|-- THIS SOFTWARE IS PROVIDED BY FREESCALE "AS IS" AND ANY EXPRESSED OR
|-- IMPLIED WARRANTIES, INCLUDING, BUT NOT LIMITED TO, THE IMPLIED WARRANTIES
|-- OF MERCHANTABILITY AND FITNESS FOR A PARTICULAR PURPOSE ARE DISCLAIMED.
|-- IN NO EVENT SHALL FREESCALE OR ITS CONTRIBUTORS BE LIABLE FOR ANY DIRECT,
|-- INDIRECT, INCIDENTAL, SPECIAL, EXEMPLARY, OR CONSEQUENTIAL DAMAGES
|-- (INCLUDING, BUT NOT LIMITED TO, PROCUREMENT OF SUBSTITUTE GOODS OR
|-- SERVICES; LOSS OF USE, DATA, OR PROFITS; OR BUSINESS INTERRUPTION)
|-- HOWEVER CAUSED AND ON ANY THEORY OF LIABILITY, WHETHER IN CONTRACT,
|-- STRICT LIABILITY, OR TORT (INCLUDING NEGLIGENCE OR OTHERWISE) ARISING
|-- IN ANY WAY OUT OF THE USE OF THIS SOFTWARE, EVEN IF ADVISED OF
|-- THE POSSIBILITY OF SUCH DAMAGE.
[IBIS Ver]   5.0
[Comment Char] |_char
[File name]   k10_120_144mbga_full.ibs
[File Rev]   1.2
[Date]   12/03/2013
[Source]   Freescale, MSG, MCD, Design
[Notes]   IBIS model for K10 microprocessor covers 1.71 - 3.6V range
[Disclaimer]   The model given below represents 144MBGA package on K10 family
[Copyright]   Copyright, Freescale, Inc., 2013
|  Component K10
[Component]   K10
[Manufacturer]  Freescale, Inc.
[Package]
|   typ   min   max
R_pkg   0.10565   0.037083   0.19461
L_pkg   2.143e-9   8.357e-10   4.07e-9
C_pkg   1.414e-12   1.006e-12   2.364e-12
[Pin]   Signal_name   model_name   R_pin   L_pin   C_pin
E5   VDD   POWER
E6   VDD   POWER
E7   VDD   POWER
E8   VDD   POWER
H5   VDDA   POWER
F5   VDD   POWER
F8   VDD   POWER
L6   VBAT   POWER
J3   ADC0SE16   NC   0.10508   2.028e-9   1.342e-12
K3   ADC1SE16   NC   0.11747   2.367e-9   1.292e-12
L3   DAC0OUT   NC   0.13114   2.72e-9   1.006e-12
L4   DAC1OUT   NC   0.15914   3.268e-9   1.044e-12
M6   EXTAL32   NC   0.12813   2.565e-9   1.428e-12
L2   PGA0DM   NC   0.14615   2.953e-9   1.472e-12
L1   PGA0DP   NC   0.15139   3.103e-9   1.367e-12
M2   PGA1DM   NC   0.19232   3.805e-9   1.477e-12
M1   PGA1DP   NC   0.19461   4.07e-9   1.434e-12
J2   PGA2DM   NC   0.11185   2.269e-9   1.308e-12
J1   PGA2DP   NC   0.1272   2.588e-9   1.118e-12
K2   PGA3DM   NC   0.14114   2.945e-9   1.334e-12
K1   PGA3DP   NC   0.15112   3.109e-9   1.208e-12
J5   PTA0   io_5vtol   0.085916   1.614e-9   1.553e-12
J6   PTA1   io_5vtol   0.080095   1.545e-9   1.48e-12
K6   PTA2   io_5vtol   0.10608   2.149e-9   1.387e-12
K7   PTA3   io_5vtol   0.083787   1.682e-9   1.243e-12
L7   PTA4   io_5vtol   0.074317   1.445e-9   1.236e-12
M8   PTA5   io_5vtol   0.11703   2.228e-9   1.217e-12
J7   PTA6   io_fast_5vtol   0.087601   1.654e-9   1.345e-12
J8   PTA7   io_fast_5vtol   0.061512   1.189e-9   1.346e-12
K8   PTA8   io_fast_5vtol   0.082315   1.601e-9   1.241e-12
L8   PTA9   io_fast_5vtol   0.082432   1.636e-9   1.26e-12
M9   PTA10   io_fast_5vtol   0.12012   2.346e-9   1.283e-12
L9   PTA11   io_fast_5vtol   0.1016   2.218e-9   1.246e-12
K9   PTA12   io_fast_5vtol   0.13102   2.548e-9   1.539e-12
J9   PTA13   io_fast_5vtol   0.082829   1.55e-9   1.505e-12
L10   PTA14   io_fast_5vtol   0.1235   2.376e-9   1.252e-12
L11   PTA15   io_fast_5vtol   0.11705   2.305e-9   1.425e-12
K10   PTA16   io_fast_5vtol   0.080134   1.565e-9   1.363e-12
K11   PTA17   io_fast_5vtol   0.10544   2.064e-9   1.471e-12
M12   PTA18   io_5vtol   0.12208   2.34e-9   1.18e-12
M11   PTA19   io_5vtol   0.1348   2.569e-9   1.539e-12
K12   PTA24   io_fast_5vtol   0.092387   1.857e-9   1.164e-12
J12   PTA25   io_fast_5vtol   0.10858   2.193e-9   1.185e-12
J11   PTA26   io_fast_5vtol   0.082775   1.67e-9   1.213e-12
J10   PTA27   io_fast_5vtol   0.075211   1.555e-9   1.137e-12
H12   PTA28   io_fast_5vtol   0.087821   1.8e-9   1.229e-12
H11   PTA29   io_fast_5vtol   0.078838   1.603e-9   1.132e-12
H10   PTB0   io_5vtol   0.076376   1.584e-9   1.092e-12
H9   PTB1   io_5vtol   0.097344   2.017e-9   1.095e-12
G12   PTB2   io_5vtol   0.117   2.368e-9   1.22e-12
G11   PTB3   io_5vtol   0.094803   1.911e-9   1.202e-12
G10   PTB4   io_5vtol   0.068112   1.419e-9   1.064e-12
G9   PTB5   io_5vtol   0.092377   1.909e-9   1.085e-12
F12   PTB6   io_5vtol   0.12901   2.639e-9   1.02e-12
F11   PTB7   io_5vtol   0.095043   1.916e-9   1.285e-12
F10   PTB8   io_5vtol   0.078152   1.654e-9   1.211e-12
F9   PTB9   io_5vtol   0.082739   1.643e-9   1.198e-12
E12   PTB10   io_5vtol   0.12458   2.568e-9   1.247e-12
E11   PTB11   io_5vtol   0.099849   1.841e-9   1.389e-12
E10   PTB16   io_5vtol   0.085079   1.669e-9   1.472e-12
E9   PTB17   io_5vtol   0.069054   1.317e-9   1.322e-12
D12   PTB18   io_5vtol   0.11503   2.345e-9   1.285e-12
D11   PTB19   io_5vtol   0.088339   1.83e-9   1.345e-12
D10   PTB20   io_5vtol   0.065585   1.375e-9   1.389e-12
D9   PTB21   io_5vtol   0.069185   1.41e-9   1.442e-12
C12   PTB22   io_5vtol   0.11404   2.464e-9   1.227e-12
C11   PTB23   io_5vtol   0.099768   2.058e-9   1.337e-12
B12   PTC0   io_5vtol   0.12229   2.5e-9   1.328e-12
B11   PTC1   io_5vtol   0.11559   2.345e-9   1.401e-12
A12   PTC2   io_5vtol   0.13984   2.835e-9   1.494e-12
A11   PTC3   io_5vtol   0.13365   2.663e-9   1.396e-12
A9   PTC4   io_5vtol   0.1265   2.554e-9   1.293e-12
D8   PTC5   io_5vtol   0.10669   2.077e-9   1.628e-12
C8   PTC6   io_5vtol   0.11206   2.413e-9   1.521e-12
B8   PTC7   io_5vtol   0.11204   2.323e-9   1.451e-12
A8   PTC8   io_5vtol   0.12537   2.609e-9   1.145e-12
D7   PTC9   io_5vtol   0.086116   1.68e-9   1.496e-12
C7   PTC10   io_5vtol   0.070007   1.465e-9   1.573e-12
B7   PTC11   io_5vtol   0.10342   2.248e-9   1.503e-12
A7   PTC12   io_5vtol   0.13637   2.826e-9   1.194e-12
D6   PTC13   io_5vtol   0.095363   1.858e-9   1.621e-12
C6   PTC14   io_5vtol   0.092937   2.013e-9   1.563e-12
B6   PTC15   io_5vtol   0.10605   2.025e-9   1.475e-12
A6   PTC16   io_5vtol   0.12921   2.609e-9   1.077e-12
D5   PTC17   io_5vtol   0.084782   1.595e-9   1.591e-12
C5   PTC18   io_5vtol   0.083266   1.685e-9   1.458e-12
B5   PTC19   io_5vtol   0.098857   1.961e-9   1.485e-12
A5   PTD0   io_5vtol   0.12572   2.617e-9   1.221e-12
D4   PTD1   io_5vtol   0.078944   1.538e-9   1.709e-12
C4   PTD2   io_5vtol   0.084711   1.875e-9   1.526e-12
B4   PTD3   io_5vtol   0.10484   2.457e-9   1.519e-12
A4   PTD4   io_5vtol   0.14437   2.961e-9   1.172e-12
A3   PTD5   io_5vtol   0.14977   3.03e-9   1.464e-12
A2   PTD6   io_5vtol   0.16664   3.369e-9   1.576e-12
A1   PTD7   io_5vtol   0.10422   2.559e-9   2.028e-12
C9   PTD8   io_5vtol   0.16612   3.291e-9   2.364e-12
B9   PTD9   io_5vtol   0.17757   3.571e-9   1.735e-12
B3   PTD10   io_5vtol   0.10564   2.157e-9   1.506e-12
B2   PTD11   io_5vtol   0.12097   2.465e-9   1.514e-12
B1   PTD12   io_5vtol   0.12863   2.642e-9   1.451e-12
C3   PTD13   io_5vtol   0.070416   1.442e-9   1.378e-12
C2   PTD14   io_5vtol   0.092443   1.923e-9   1.425e-12
C1   PTD15   io_5vtol   0.12495   2.75e-9   1.349e-12
D3   PTE0   io_5vtol   0.084602   1.668e-9   1.402e-12
D2   PTE1   io_5vtol   0.089226   1.735e-9   1.422e-12
D1   PTE2   io_5vtol   0.083503   1.676e-9   1.529e-12
E4   PTE3   io_5vtol   0.08506   1.514e-9   1.429e-12
E3   PTE4   io_5vtol   0.070373   1.35e-9   1.319e-12
E2   PTE5   io_5vtol   0.081005   1.704e-9   1.587e-12
E1   PTE6   io_5vtol   0.10882   2.322e-9   1.357e-12
F4   PTE7   io_5vtol   0.081476   1.563e-9   1.401e-12
F3   PTE8   io_5vtol   0.10261   1.98e-9   1.406e-12
F2   PTE9   io_5vtol   0.090294   1.774e-9   1.431e-12
F1   PTE10   io_5vtol   0.12893   2.553e-9   1.396e-12
G4   PTE11   io_5vtol   0.082172   1.716e-9   1.349e-12
G3   PTE12   io_5vtol   0.1099   2.197e-9   1.371e-12
H1   PTE16   io_5vtol   0.098212   1.973e-9   1.744e-12
H2   PTE17   io_5vtol   0.095025   1.855e-9   2.056e-12
G1   PTE18   io_5vtol   0.045567   1.064e-9   1.682e-12
G2   PTE19   io_5vtol   0.037083   8.357e-10   1.78e-12
M4   PTE24   io_5vtol   0.077072   1.569e-9   1.901e-12
K5   PTE25   io_5vtol   0.053437   1.114e-9   1.764e-12
K4   PTE26   io_5vtol   0.060417   1.149e-9   1.778e-12
J4   PTE27   io_5vtol   0.077191   1.564e-9   2.165e-12
H4   PTE28   io_5vtol   0.074786   1.53e-9   2.253e-12
L12   RESETB   io_3v   0.061938   1.604e-9   1.471e-12
L5   RTC_WAKEUP_B   io_3v   0.13699   3.096e-9   1.167e-12
G5   VREFH   NC   0.17633   3.372e-9   1.772e-12
G6   VREFL   NC   0.19035   3.548e-9   1.71e-12
M3   VREFOUT   NC   0.17093   3.542e-9   1.243e-12
M7   XTAL32   NC   0.1497   2.904e-9   1.345e-12
F6   VSS   GND
F7   VSS   GND
G7   VSS   GND
G8   VSS   GND
H3   VSS   GND
H7   VSS   GND
H8   VSS   GND
M10   VSS   GND
H6   VSSA   GND
|End [Component]
[Component] io65u65dgo6m3v
|   Component io65u65dgo6m3v
| This component was characterised for following simulation conditions:
| Temperature:
|   - Typ: 25.0C,   - Min: 125.0C,   - Max: -40.0C
| External (pad) voltage:
|   - Typ: 3.3V,   - Min: 1.71V,   - Max: 3.6V
| Internal (core) voltage:
|   - Typ: 3.3V,   - Min: 1.71V,   - Max: 3.6V
[Manufacturer] Freescale Semiconductor
[Package]
| variable   typ   min   max
R_pkg   0.2240   0.2240   0.2240
L_pkg   8.5100nH   8.5100nH   8.5100nH
C_pkg   0.2740pF   0.2740pF   0.2740pF
[Pin]  signal_name   model_name   R_pin   L_pin   C_pin
fpad   pad   io_3v_trig
pad   pad   io_3v
vdd3v  vdd3v   POWER
vss3v  vss3v   GND
|obe   obe   dummy
|do   do   dummy
[Model Selector] io_3v_trig
io_3v_trig_dse1_sre0   io with trigger, full drive mode without slew rate
io_3v_trig_dse1_sre1   io with trigger, full drive mode with slew rate
io_3v_trig_dse0_sre0   io with trigger, low drive mode without slew rate
io_3v_trig_dse0_sre1   io with trigger, low drive mode with slew rate
[Model Selector] io_3v
io_3v_dse1_sre0   io, full drive mode without slew rate
io_3v_dse1_sre1   io, full drive mode with slew rate
io_3v_dse0_sre0   io, low drive mode without slew rate
io_3v_dse0_sre1   io, low drive mode with slew rate
[Component] io80u65dgo6m5vtol
|   Component io80u65dgo6m5vtol
| This component was characterised for following simulation conditions:
| Spice Models:
|  - Typ Condition
|   /proj/tec16/analog/modules/IO_C90/io80u65dgo4m5vtol/users/antony/ibis/io80u/6m1t/cmos090sgtfs_typ.model
|  - Min Condition
|   /proj/tec16/analog/modules/IO_C90/io80u65dgo4m5vtol/users/antony/ibis/io80u/6m1t/cmos090sgtfs_wcs.model
|  - Max Condition
|   /proj/tec16/analog/modules/IO_C90/io80u65dgo4m5vtol/users/antony/ibis/io80u/6m1t/cmos090sgtfs_bcs.model
| Spice  Netlist:
|  - Typ Condition
|   /proj/tec16/analog/modules/IO_C90/io80u65dgo4m5vtol/users/antony/ibis/io80u/6m1t/io.ckt
|  - Min Condition
|   /proj/tec16/analog/modules/IO_C90/io80u65dgo4m5vtol/users/antony/ibis/io80u/6m1t/io.ckt
|  - Max Condition
|   /proj/tec16/analog/modules/IO_C90/io80u65dgo4m5vtol/users/antony/ibis/io80u/6m1t/io.ckt
| Temperature:
|   - Typ: 25.0C,   - Min: 125.0C,   - Max: -40.0C
| External (pad) voltage:
|   - Typ: 3.3V,   - Min: 1.71V,   - Max: 3.6V
| Internal (core) voltage:
|   - Typ: 1.2V,   - Min: 1.08V,   - Max: 1.32V
[Manufacturer] Freescale Semiconductor
[Package]
| variable   typ   min   max
R_pkg   0.2240   0.2240   0.2240
L_pkg   8.5100nH   8.5100nH   8.5100nH
C_pkg   0.2740pF   0.2740pF   0.2740pF
[Pin]  signal_name   model_name   R_pin   L_pin   C_pin
fpad   pad   io_fast_5vtol
pad   pad   io_5vtol
|vsslv vsslv   iGND
|vddlv vddlv   iPOWER
vdd3v  vdd3v   POWER
vss3v  vss3v   GND
|obe   obe   dummy
|do   do   dummy
[Model Selector] io_fast_5vtol
io_fast_5vtol_dse1_sre0   fast io, full drive mode without slew rate
io_fast_5vtol_dse1_sre1   fast io, full drive mode with slew rate
io_fast_5vtol_dse0_sre0   fast io, low drive mode without slew rate
io_fast_5vtol_dse0_sre1   fast io, low drive mode with slew rate
[Model Selector] io_5vtol
io_5vtol_dse1_sre0   io, full drive mode without slew rate
io_5vtol_dse1_sre1   io, full drive mode with slew rate
io_5vtol_dse0_sre0   io, low drive mode without slew rate
io_5vtol_dse0_sre1   io, low drive mode with slew rate
| Models and submodels in the file (16): io_3v_trig_dse1_sre0 (I/O), io_3v_dse1_sre0 (I/O), io_3v_trig_dse1_sre1 (I/O), io_3v_dse1_sre1 (I/O), io_3v_trig_dse0_sre0 (I/O), io_3v_dse0_sre0 (I/O), io_3v_trig_dse0_sre1 (I/O), io_3v_dse0_sre1 (I/O), io_fast_5vtol_dse1_sre0 (I/O), io_5vtol_dse1_sre0 (I/O), io_fast_5vtol_dse1_sre1 (I/O), io_5vtol_dse1_sre1 (I/O), io_fast_5vtol_dse0_sre0 (I/O), io_5vtol_dse0_sre0 (I/O), io_fast_5vtol_dse0_sre1 (I/O), io_5vtol_dse0_sre1 (I/O)
